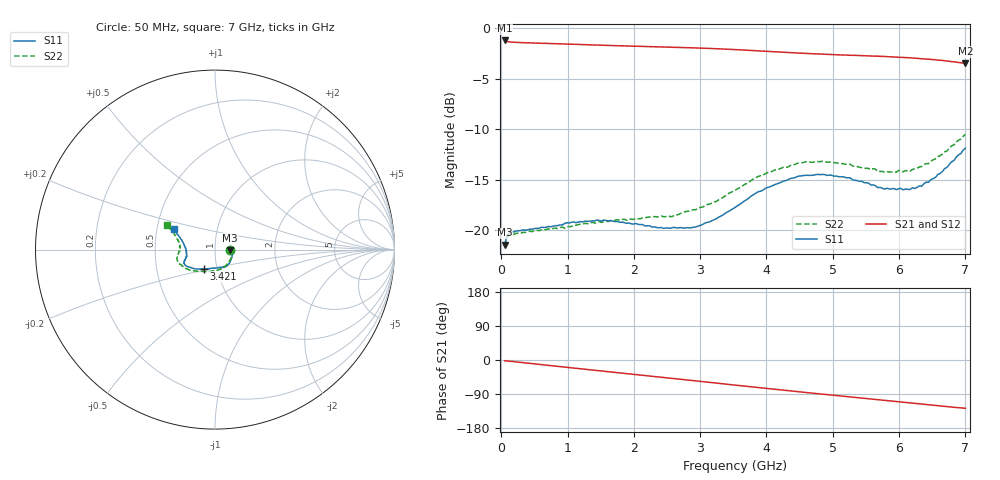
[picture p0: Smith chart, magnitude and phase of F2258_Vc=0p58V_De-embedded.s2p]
! Integrated Device Technology
! Corporate Headquarters
! 6024 Silver Creek Valley Road
! San Jose, CA 95138  USA
! Phone:  1-408-284-8200
! Toll Free:  1-800-223-1366
! Webpage:  http://www.idt.com/
! Timing and RF Division
! 515 Groton Road, Suite 102
! Westford, MA 01886-6024
! Device:  F2258
! Description: Voltage Variable RF Attenuator
! Frequency:  50.0 -  6000.00 MHz
! Package:  3x3 mm Thin QFN Plastic Package: 16 pin
! Ports:  2 RF, 2 DC
!  Pin  1  = NC
!  Pin  2  = NC
!  Pin  3  = RF2  = Port 2
!  Pin  4  = GND
!  Pin  5  = Vdd
!  Pin  6  = NC
!  Pin  7  = VCTRL
!  Pin  8  = NC
!  Pin  9  = GND
!  Pin 10  = RF1  = Port 1
!  Pin 11  = NC
!  Pin 12  = NC
!  Pin 13  = NC
!  Pin 14  = NC
!  Pin 15  = NC
!  Pin 16  = NC
! Vcntrl:  0.580 Volts
! Vdd:  +3.300 Volts
! Current:  1.107 mA
! Data:  The device was measured on a the F2258 evaluation board which has
!  individual transmission lines to the RF pins.  Data was collected
!  using a calibrated network analyzer.  The evaluation board was
!  de-embedded using a TRL calibration technique.
!  The reference plane is the edge of the package pin.
! Misc:  SN 10
!  Action Tracker AT0285
! Date Measured:  2014-12-10
! Date:  2016-01-13  MJV
! Note:
!  Integrated Device Technology supplies this data as a sample of measured
!  data at the package pin for this product.  Your particular data for this
!  product may vary.
!  Data was taken at 25 degrees C.
!  Integrated Device Technology reserves the right to change this data at anytime.
!Freq_(GHz)  S11M_(dB)  S11P_(deg)  S21M_(dB)  S21P_(deg)  S12M_(dB)  S12P_(deg)  S22M_(dB)  S22P_(deg)
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# GHz S dB R 50
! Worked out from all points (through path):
!   201 points, 50 MHz to 7 GHz, reference 50 ohm
!   highest |S21| = -1.23 dB at 50 MHz (marker M1); lowest = -3.5 dB at 7 GHz (marker M2)
!   group delay of S21, straight-line fit = 50.5 ps
!   lowest |S11| = -21.4 dB at 50 MHz (marker M3), VSWR 1.19, Z = 59.3 - j0.491 ohm
!   |S11| at or under -10 dB: start of sweep to end of sweep
!   |S22| runs from -21.6 to -10.5 dB; largest |S21 - S12| = 0.00059
!   S11 on the Smith chart (normalised r, x): 50 MHz: 1.19, -0.01; 3.421 GHz: 0.87, -0.19; 7 GHz: 0.61, +0.15
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0.05  -21.42 -2.8  -1.23 -2.0  -1.23 -2.0  -21.56 -2.8
0.08475  -20.55 -4.4  -1.32 -2.5  -1.33 -2.5  -20.71 -4.6
0.15425  -20.14 -6.9  -1.39 -3.7  -1.39 -3.7  -20.39 -8.0
0.745  -19.64 -30.3  -1.53 -14.8  -1.54 -14.8  -19.89 -35.3
1.2315  -19.15 -47.5  -1.64 -23.9  -1.64 -23.9  -19.38 -56.0
1.6485  -19.01 -58.0  -1.72 -31.5  -1.73 -31.5  -19.04 -69.0
2.37825  -19.74 -75.9  -1.86 -44.8  -1.86 -44.8  -18.65 -88.0
2.58675  -19.71 -82.4  -1.90 -48.6  -1.90 -48.6  -18.60 -94.6
2.93425  -19.66 -97.2  -1.97 -55.1  -1.97 -55.1  -17.95 -107.0
3.247  -18.84 -111.3  -2.04 -61.0  -2.05 -61.0  -17.12 -119.4
3.42075  -18.15 -119.7  -2.10 -64.3  -2.10 -64.3  -16.39 -126.6
3.525  -17.74 -123.7  -2.13 -66.2  -2.13 -66.2  -16.04 -130.5
4.0115  -15.77 -140.5  -2.30 -75.3  -2.31 -75.3  -14.29 -146.9
4.46325  -14.68 -150.2  -2.47 -83.4  -2.47 -83.4  -13.37 -158.5
4.7065  -14.54 -153.6  -2.54 -87.7  -2.55 -87.7  -13.26 -163.0
5.2625  -14.81 -160.1  -2.70 -97.4  -2.70 -97.4  -13.46 -171.6
5.6795  -15.78 -165.8  -2.78 -104.6  -2.78 -104.6  -14.18 -177.4
5.85325  -15.91 -169.9  -2.84 -107.7  -2.84 -107.7  -14.21 177.9
6.166  -15.95 -178.0  -2.94 -113.3  -2.94 -113.3  -14.15 171.6
6.33975  -15.64 175.0  -3.03 -116.4  -3.02 -116.4  -13.68 167.1
6.6525  -14.19 163.6  -3.20 -121.9  -3.20 -121.9  -12.46 160.1
7  -11.87 153.9  -3.50 -127.4  -3.50 -127.4  -10.51 152.5
